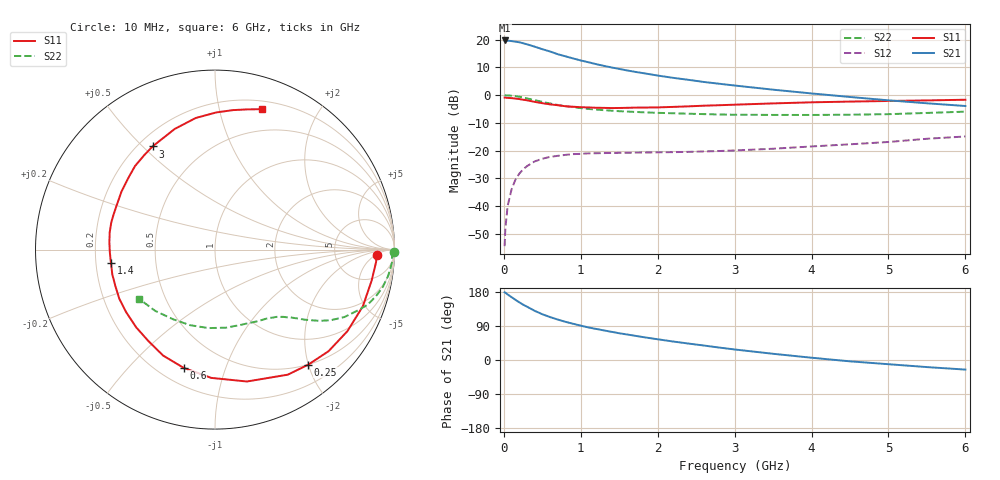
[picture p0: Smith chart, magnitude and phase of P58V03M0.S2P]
! SIEMENS Small Signal Semiconductors
! BFP183
! Si NPN RF Bipolar Junction Transistor in SOT143
! VCE = 8 V  IC = 3 mA
! Common Emitter S-Parameters:  March  1996
# GHz  S  MA  R  50
!  f  S11  S21  S12  S22
! GHz  MAG  ANG  MAG  ANG  MAG  ANG  MAG  ANG
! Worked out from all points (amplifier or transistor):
!   36 points, 10 MHz to 6 GHz, reference 50 ohm
!   highest |S21| = 19.7 dB at 10 MHz (marker M1)
!   |S21| within 3 dB of that: start of sweep to 484.4 MHz
!   unconditionally stable (mu >= 1): 1.939 GHz to 5.783 GHz
!   at 250 MHz: K = 0.15, MSG = 22.7 dB, |S12| = -26.8 dB
!   at 1.4 GHz: K = 0.77, MSG = 15.4 dB, |S12| = -20.8 dB
!   at 6 GHz: K = 0.96, MSG = 5.5 dB, |S12| = -14.9 dB
!   lowest NFmin = 1.10 dB at 450 MHz
!   S11 on the Smith chart (normalised r, x): 10 MHz: 17, -6; 250 MHz: 0.50, -2.00; 600 MHz: 0.30, -0.73; 1.4 GHz: 0.26, -0.06; 3 GHz: 0.26, +0.54; 6 GHz: 0.28, +1.35
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0.01  0.9007 -2.0  9.643 178.7  0.0019 82.0  0.9969 -0.8
0.02  0.9002 -4.4  9.626 177.6  0.004 89.0  0.9866 -1.7
0.05  0.8898 -11.1  9.555 172.8  0.0102 85.1  0.9886 -4.2
0.1  0.8823 -20.9  9.398 165.9  0.0199 78.3  0.9761 -8.5
0.2  0.849 -41.8  8.951 152.3  0.0383 67.9  0.9338 -16.1
0.25  0.8251 -51.0  8.592 146.1  0.0458 62.8  0.9056 -19.7
0.3  0.8063 -59.8  8.229 140.8  0.0524 58.3  0.8721 -22.5
0.4  0.7561 -76.4  7.459 129.9  0.0638 50.3  0.8135 -27.5
0.5  0.715 -91.7  6.716 120.8  0.0714 43.7  0.7567 -31.3
0.6  0.6813 -104.9  6.109 113.3  0.0771 38.6  0.7062 -34.2
0.7  0.6573 -116.1  5.453 106.8  0.0805 34.9  0.6649 -36.3
0.8  0.6302 -126.1  4.999 100.8  0.0838 31.4  0.6327 -38.1
0.9  0.6168 -135.4  4.578 95.6  0.0864 28.9  0.6061 -39.4
1.1  0.5995 -152.7  3.906 85.9  0.0893 25.0  0.5627 -42.1
1.4  0.5844 -172.9  3.15 74.4  0.0907 21.4  0.5237 -45.7
1.8  0.5974 165.4  2.499 60.8  0.0925 19.6  0.4906 -50.7
2.2  0.613 148.3  2.046 48.8  0.0938 19.4  0.4706 -56.6
3  0.6718 121.2  1.488 27.8  0.1006 22.1  0.4431 -71.3
3.5  0.7086 108.5  1.252 16.4  0.1081 23.9  0.4394 -82.0
4.5  0.7642 89.5  0.925 -3.5  0.1299 24.8  0.4437 -108.5
5.5  0.8022 76.9  0.712 -18.7  0.1635 23.0  0.4772 -134.4
6  0.8248 71.5  0.636 -25.3  0.1798 19.6  0.5033 -146.8
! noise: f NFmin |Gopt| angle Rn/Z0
0.45  1.1  0.37  35  0.3
0.9  1.15  0.34  85  0.23
1.8  1.9  0.35  160  0.13
